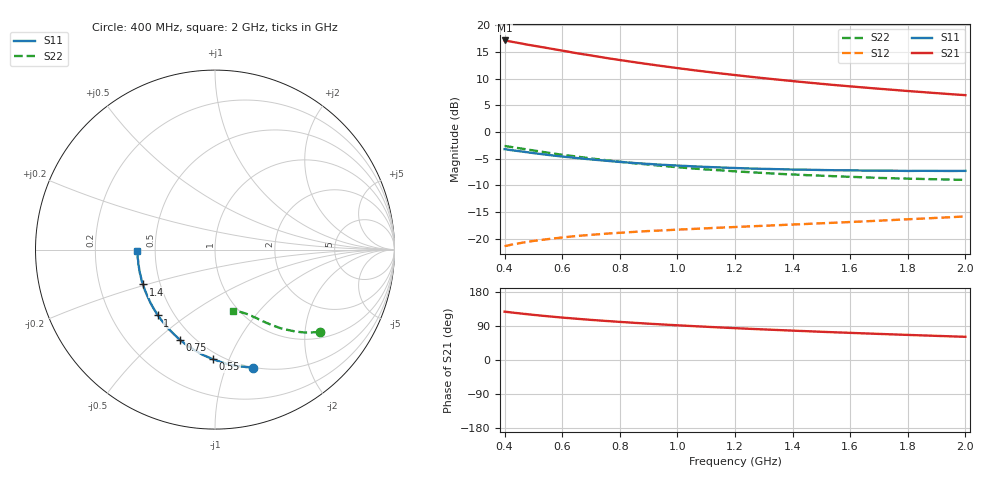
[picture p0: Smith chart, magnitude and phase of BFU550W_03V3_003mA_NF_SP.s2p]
! Filename:  P:\Prog\Test\Noise\ATS_data\Testdata_Net\06 Compressed Noise after Statistics\BFU550W_APM2013_11_D05_03p3V_003mA_NF_CM01_D.sf
! Date/Time: Tue 26/Mar/2013 16:25:27
! BFU550W_APM2013_11_D05_03p3V_1to35mA_NF_CM01_Bias3_R.sf
! Noise Parameter Data File
! BFU550W_APM2013_11_D05_03p3V_1to35mA_NF_CM01
! Date/time: Mon Mar 25 12:16:07 2013
! VAR V_out= 3.300000
! VAR I_out= 2.990000
! VAR V_in= 0.803100
! VAR I_in= 0.031110
! Device data file deembeded for feedlines and parallel
! Original file: \06 Compressed Noise after Statistics\BFU550W_APM2013_11_D05_03p3V_003mA_NF_CM01_R.sf
! Feed-files: PR019V01_070313_Feed1.s2p, PR019V01_070313_Feed2.s2p
! Parallel-file: PR019V01_070313_Par.s2p
# MHz S MA R 50
!  Freq-MHz  S11-mag  S11-arg  S21-mag  S21-arg  S12-mag  S12-arg  S22-mag  S22-arg
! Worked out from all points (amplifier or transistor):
!   37 points, 400 MHz to 2 GHz, reference 50 ohm
!   highest |S21| = 17.1 dB at 400 MHz (marker M1)
!   |S21| within 3 dB of that: start of sweep to 721.7 MHz
!   unconditionally stable (mu >= 1): 1.911 GHz to end of sweep
!   at 500 MHz: K = 0.37, MSG = 18.3 dB, |S12| = -20.4 dB
!   at 1.1 GHz: K = 0.73, MSG = 14.7 dB, |S12| = -18.0 dB
!   at 2 GHz: K = 1.01, MAG = 10.6 dB, |S12| = -15.8 dB
!   lowest NFmin = 0.51 dB at 420 MHz
!   S11 on the Smith chart (normalised r, x): 400 MHz: 0.50, -1.25; 550 MHz: 0.45, -0.87; 750 MHz: 0.42, -0.60; 1 GHz: 0.41, -0.39; 1.4 GHz: 0.40, -0.19; 2 GHz: 0.40, -0.01
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400  0.6906 -72.0  7.187 127.6  0.0855 54.4  0.7406 -38.1
420  0.6785 -74.9  7.033 125.8  0.08784 53.4  0.7265 -39.3
440  0.6676 -77.6  6.875 124.0  0.09004 52.4  0.7125 -40.4
480  0.646 -82.7  6.562 120.8  0.09389 50.8  0.6855 -42.4
500  0.6351 -85.3  6.425 119.1  0.09571 50.0  0.6723 -43.3
550  0.6107 -91.1  6.093 115.4  0.09953 48.4  0.6407 -45.5
600  0.5899 -96.8  5.774 111.9  0.1031 47.0  0.6126 -47.2
650  0.5711 -101.7  5.465 108.9  0.1064 45.9  0.5895 -48.9
700  0.5541 -106.8  5.202 105.9  0.1091 45.0  0.5658 -50.5
750  0.5394 -111.3  4.944 103.2  0.1118 44.3  0.5457 -51.7
800  0.5248 -115.7  4.716 100.6  0.1141 43.7  0.5272 -53.0
850  0.5129 -119.9  4.505 98.1  0.1163 43.2  0.5101 -54.1
950  0.4931 -127.3  4.129 93.7  0.1202 42.7  0.4809 -56.2
1000  0.4856 -130.9  3.963 91.6  0.1221 42.6  0.4686 -57.0
1100  0.4716 -137.4  3.666 87.7  0.1256 42.6  0.4464 -58.8
1200  0.4604 -143.4  3.412 84.1  0.1292 42.8  0.4288 -60.5
1300  0.4522 -149.1  3.189 80.7  0.1326 43.2  0.4135 -62.1
1400  0.4456 -154.2  2.995 77.5  0.1362 43.8  0.4009 -63.5
1500  0.441 -159.0  2.824 74.5  0.14 44.5  0.3902 -65.2
1600  0.438 -163.6  2.674 71.6  0.1439 45.2  0.3808 -66.8
1750  0.4346 -169.7  2.479 67.5  0.1503 46.5  0.3688 -69.1
2000  0.4328 -179.2  2.213 61.2  0.1623 48.5  0.3564 -73.4
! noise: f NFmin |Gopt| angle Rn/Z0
400  0.5179  0.3474  34.33  0.13
460  0.535  0.3388  41.9  0.1272
600  0.5561  0.3232  45.96  0.1421
800  0.6132  0.3418  68.77  0.114
1000  0.6902  0.3477  79.22  0.1143
1200  0.6962  0.3566  97.73  0.1026
1400  0.7557  0.3691  113.2  0.0896
1600  0.7135  0.3671  126.8  0.0819
1800  0.8596  0.388  140.5  0.0694
2000  0.8844  0.363  159.3  0.0694
